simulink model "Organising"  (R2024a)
settings: Solver=VariableStepAuto  StartTime=0.0  StopTime=10.0  RelTol=1e-3
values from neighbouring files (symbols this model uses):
  b = 0.10    (= 0.1)    [InitMotor.m]
  J = 0.01    [InitMotor.m]
  K = 0.01    [InitMotor.m]
  L = 0.50    (= 0.5)    [InitMotor.m]
undefined symbols (not defined in the file or in its folder): R

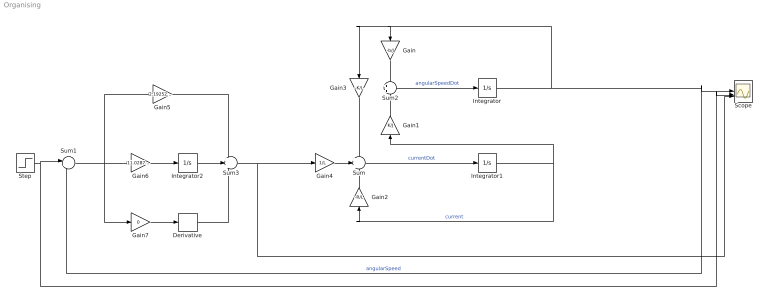
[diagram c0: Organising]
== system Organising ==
  Derivative : Derivative
  Gain : Gain  Gain=-b/J
  Gain1 : Gain  Gain=K/J
  Gain2 : Gain  Gain=-R/L
  Gain3 : Gain  Gain=-K/L
  Gain4 : Gain  Gain=1/L
  Gain5 : Gain  Gain=2.19252511826487
  Gain6 : Gain  Gain=11.0287321848786
  Gain7 : Gain  Gain=0
  Integrator : Integrator
  Integrator1 : Integrator
  Integrator2 : Integrator
  Scope : Scope  NumInputPorts=3
  Step : Step  SampleTime=0
  Sum : Sum  Inputs=+++
  Sum1 : Sum  Inputs=|+-
  Sum2 : Sum  Inputs=+|+
  Sum3 : Sum  Inputs=+++
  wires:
  Integrator/1 -> Sum1/2, Scope/1, Gain3/1, Gain/1  "angularSpeed"
  Integrator1/1 -> Gain2/1, Gain1/1  "current"
  Sum2/1 -> Integrator/1  "angularSpeedDot"
  Sum/1 -> Integrator1/1  "currentDot"
  Gain/1 -> Sum2/1
  Gain1/1 -> Sum2/2
  Gain2/1 -> Sum/3
  Gain3/1 -> Sum/1
  Gain4/1 -> Sum/2
  Step/1 -> Scope/2, Sum1/1
  Gain6/1 -> Integrator2/1
  Gain5/1 -> Sum3/1
  Sum3/1 -> Scope/3, Gain4/1
  Gain7/1 -> Derivative/1
  Integrator2/1 -> Sum3/2
  Sum1/1 -> Gain7/1, Gain5/1, Gain6/1
  Derivative/1 -> Sum3/3
